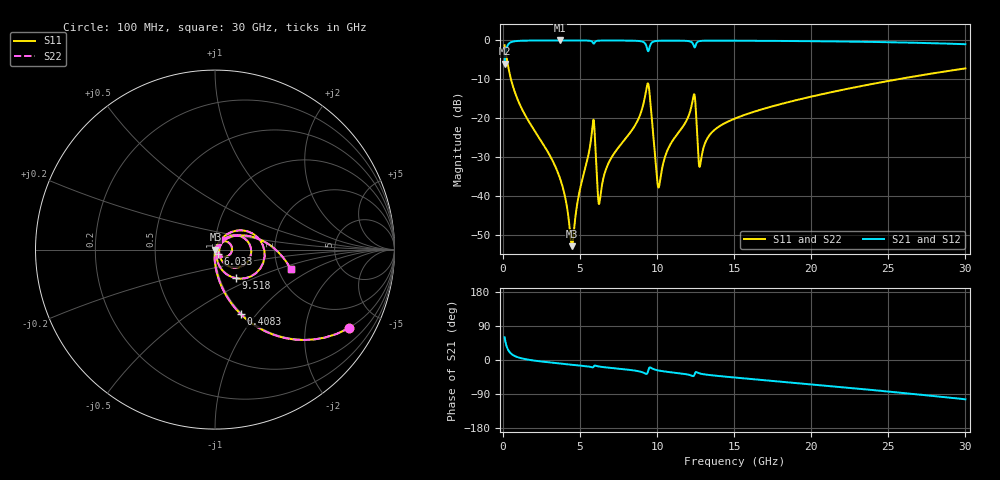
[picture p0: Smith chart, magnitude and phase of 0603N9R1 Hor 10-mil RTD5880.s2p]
# GHz S MA R 50
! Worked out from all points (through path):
!   3201 points, 100 MHz to 30 GHz, reference 50 ohm
!   highest |S21| = -0.02 dB at 3.707 GHz (marker M1); lowest = -6.0 dB at 100 MHz (marker M2)
!   group delay of S21, straight-line fit = 10.1 ps
!   lowest |S11| = -52.9 dB at 4.473 GHz (marker M3), VSWR 1.00, Z = 50.2 - j0.0473 ohm
!   |S11| at or under -10 dB: 514.3 MHz to 25.62 GHz (25.11 GHz wide, 192 % of centre)
!   |S22| runs from -52.9 to -1.2 dB; largest |S21 - S12| = 0
!   S11 on the Smith chart (normalised r, x): 100 MHz: 0.98, -3.44; 408.3 MHz: 0.98, -0.84; 6.033 GHz: 1.03, -0.05; 9.518 GHz: 1.19, -0.39; 30 GHz: 2.34, -0.63
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0.1  0.8662 -30.2  0.4994 59.8  0.4994 59.8  0.8662 -30.2
0.4083438  0.3885 -68.2  0.9209 21.7  0.9209 21.7  0.3885 -68.2
1.314688  0.121 -86.2  0.9916 3.3  0.9916 3.3  0.121 -86.2
3.706688  0.01653 -92.6  0.9979 -9.2  0.9979 -9.2  0.01653 -92.6
4.472875  0.002253 -12.1  0.9977 -12.3  0.9977 -12.3  0.002253 -12.1
5.089563  0.01473 63.6  0.9969 -14.8  0.9969 -14.8  0.01473 63.6
5.809031  0.0809 32.3  0.948 -19.6  0.948 -19.6  0.0809 32.3
6.033281  0.02898 -55.4  0.9775 -15.5  0.9775 -15.5  0.02898 -55.4
6.164094  0.00966 -29.8  0.9905 -16.8  0.9905 -16.8  0.00966 -29.8
6.285563  0.008981 29.1  0.9937 -17.6  0.9937 -17.6  0.008981 29.1
6.846188  0.02642 61.9  0.996 -20.2  0.996 -20.2  0.02642 61.9
9.135406  0.161 41.0  0.9458 -33.9  0.9458 -33.9  0.161 41.0
9.359656  0.2717 2.2  0.7698 -35.0  0.7698 -35.0  0.2717 2.2
9.5185  0.1966 -54.1  0.8317 -19.6  0.8317 -19.6  0.1966 -54.1
10.06978  0.01287 -19.8  0.9871 -27.5  0.9871 -27.5  0.01287 -19.8
12.33097  0.182 17.6  0.8968 -42.5  0.8968 -42.5  0.182 17.6
12.79816  0.02547 13.2  0.9829 -35.8  0.9829 -35.8  0.02547 13.2
13.47091  0.06309 44.8  0.9922 -40.1  0.9922 -40.1  0.06309 44.8
15.05  0.09886 41.2  0.9906 -46.3  0.9906 -46.3  0.09886 41.2
20.03956  0.1899 24.2  0.9767 -64.4  0.9767 -64.4  0.1899 24.2
25.01978  0.3011 5.6  0.9475 -83.3  0.9475 -83.3  0.3011 5.6
30  0.4361 -14.5  0.8928 -103.7  0.8928 -103.7  0.4361 -14.5
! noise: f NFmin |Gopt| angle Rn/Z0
0.1  0.0003234  0.9263  0.5676  0.0009733
3.417  0.003683  0.7936  9.421  0.003659
6.743  0.007377  0.7971  18.43  0.007332
10.06  0.01685  0.8635  27.41  0.02502
13.39  0.0131  0.779  36.14  0.01099
16.7  0.01261  0.725  44.52  0.007831
20.03  0.01454  0.7184  52.8  0.008248
23.35  0.01668  0.7176  60.84  0.008768
26.67  0.01901  0.7202  68.69  0.009287
30  0.02156  0.7254  76.32  0.009791
